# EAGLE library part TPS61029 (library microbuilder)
TPS61029 - Boost Converter Input: 0.9-6.5V Quiescent Current: 25uA (Typ.) TPS61029DRCT = 1.8-5.5V Output TPS61027DRCR = 5.0V Output
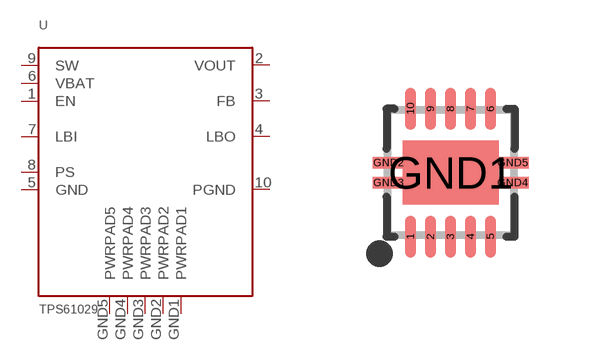
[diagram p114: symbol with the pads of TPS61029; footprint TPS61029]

Designator prefix U

## TPS61029  [TPS61029]
1  EN
2  VOUT
3  FB
4  LBO
5  GND
6  VBAT
7  LBI
8  PS
9  SW
10  PGND
GND1  PWRPAD1
GND2  PWRPAD2
GND3  PWRPAD3
GND4  PWRPAD4
GND5  PWRPAD5

## Footprint TPS61029 (pad centres in mm)
smd 0.28 x 1.05: 1 -1,-1.6; 2 -0.5,-1.6; 3 0,-1.6; 4 0.5,-1.6; 5 1,-1.6; 6 1,1.6; 7 0.5,1.6; 8 0,1.6; 9 -0.5,1.6; 10 -1,1.6
smd 2.4 x 1.6: GND1 0,0
smd 0.8 x 0.28: GND2 -1.55,0.25; GND3 -1.55,-0.25; GND4 1.55,-0.25; GND5 1.55,0.25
